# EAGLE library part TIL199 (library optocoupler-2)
TEXAS INSTRUMENTS OPTO COUPLER
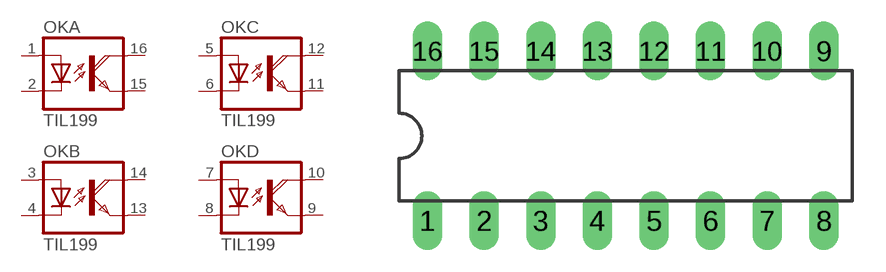
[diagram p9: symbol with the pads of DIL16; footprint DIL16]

Designator prefix OK; gates A=OK-D B=OK-D C=OK-D D=OK-D

## TIL199  [DIL16]
1  A:A  pas
2  A:C  pas
3  B:A  pas
4  B:C  pas
5  C:A  pas
6  C:C  pas
7  D:A  pas
8  D:C  pas
9  D:EMI  pas
10  D:COL  pas
11  C:EMI  pas
12  C:COL  pas
13  B:EMI  pas
14  B:COL  pas
15  A:EMI  pas
16  A:COL  pas

## Footprint DIL16 (pad centres in mm)
Dual In Line Package
drill 0.813 long: 1 -8.89,-3.81; 2 -6.35,-3.81; 3 -3.81,-3.81; 4 -1.27,-3.81; 5 1.27,-3.81; 6 3.81,-3.81; 7 6.35,-3.81; 8 8.89,-3.81; 9 8.89,3.81; 10 6.35,3.81; 11 3.81,3.81; 12 1.27,3.81; 13 -1.27,3.81; 14 -3.81,3.81; 15 -6.35,3.81; 16 -8.89,3.81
